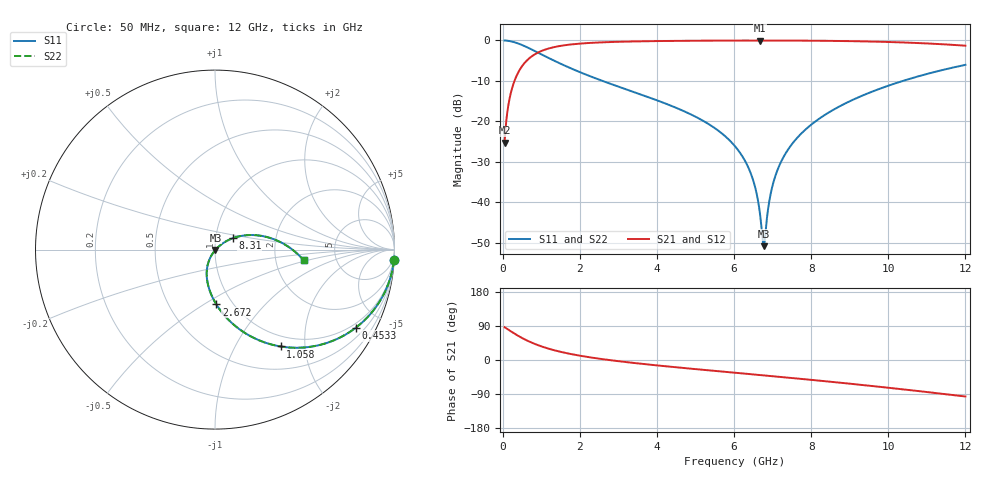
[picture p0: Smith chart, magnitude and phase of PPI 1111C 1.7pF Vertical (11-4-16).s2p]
# GHz S MA R 50
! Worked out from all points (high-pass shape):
!   1601 points, 50 MHz to 12 GHz, reference 50 ohm
!   highest |S21| = -0.03 dB at 6.675 GHz (marker M1); lowest = -25.3 dB at 50 MHz (marker M2)
!   |S21| within 3 dB of the highest: 911.2 MHz to end of sweep
!   lowest |S11| = -50.9 dB at 6.772 GHz (marker M3), VSWR 1.01, Z = 50.2 - j0.18 ohm
!   |S11| at or under -10 dB: 2.585 GHz to 10.38 GHz (7.799 GHz wide, 120 % of centre)
!   |S22| runs from -50.9 to 0.0 dB; largest |S21 - S12| = 0
!   S11 on the Smith chart (normalised r, x): 50 MHz: 1, -33; 453.3 MHz: 0.83, -3.68; 1.058 GHz: 0.83, -1.56; 2.672 GHz: 0.84, -0.57; 8.31 GHz: 1.21, +0.15; 12 GHz: 2.91, -0.47
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0.05  0.9985 -3.4  0.0543 86.6  0.0543 86.6  0.9985 -3.4
0.2143125  0.9738 -14.5  0.2271 75.5  0.2271 75.5  0.9738 -14.5
0.4533125  0.8965 -29.1  0.4426 60.9  0.4426 60.9  0.8965 -29.1
1.058281  0.6523 -55.9  0.7571 34.1  0.7571 34.1  0.6523 -55.9
2.044156  0.3976 -79.2  0.9161 10.6  0.9161 10.6  0.3976 -79.2
2.671531  0.3054 -88.6  0.9506 1.1  0.9506 1.1  0.3054 -88.6
4.038312  0.179 -104.0  0.9817 -14.6  0.9817 -14.6  0.179 -104.0
5.270656  0.09685 -115.2  0.9927 -26.6  0.9927 -26.6  0.09685 -115.2
6.025  0.04918 -120.6  0.9959 -33.6  0.9959 -33.6  0.04918 -120.6
6.450719  0.02163 -120.3  0.9967 -37.6  0.9967 -37.6  0.02163 -120.3
6.577687  0.01331 -116.7  0.9968 -38.8  0.9968 -38.8  0.01331 -116.7
6.674781  0.00708 -106.2  0.9968 -39.7  0.9968 -39.7  0.00708 -106.2
6.734531  0.003752 -81.0  0.9968 -40.2  0.9968 -40.2  0.003752 -81.0
6.771875  0.002861 -38.7  0.9968 -40.6  0.9968 -40.6  0.002861 -38.7
6.809219  0.003908 1.7  0.9967 -40.9  0.9967 -40.9  0.003908 1.7
6.966062  0.0138 35.3  0.9966 -42.4  0.9966 -42.4  0.0138 35.3
7.167719  0.02789 39.4  0.9962 -44.3  0.9962 -44.3  0.02789 39.4
7.511281  0.05294 38.9  0.995 -47.6  0.995 -47.6  0.05294 38.9
8.019156  0.09228 35.3  0.9919 -52.6  0.9919 -52.6  0.09228 35.3
8.310438  0.1162 32.8  0.9892 -55.4  0.9892 -55.4  0.1162 32.8
10.01331  0.2768 15.7  0.9559 -73.3  0.9559 -73.3  0.2768 15.7
12  0.4988 -6.9  0.8605 -96.3  0.8605 -96.3  0.4988 -6.9
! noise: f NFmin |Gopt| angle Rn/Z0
0.05  0.0006804  0.9497  2.451  0.003035
1.372  0.00399  0.6948  11.19  0.002528
2.701  0.006413  0.6399  18.69  0.003277
4.031  0.008615  0.614  26.16  0.003947
5.36  0.01076  0.6036  33.35  0.004625
6.682  0.01294  0.6038  40.14  0.005365
8.012  0.01526  0.6123  46.57  0.006229
9.341  0.01777  0.6274  52.62  0.007274
10.67  0.02058  0.648  58.3  0.008583
12  0.0238  0.673  63.68  0.01027
